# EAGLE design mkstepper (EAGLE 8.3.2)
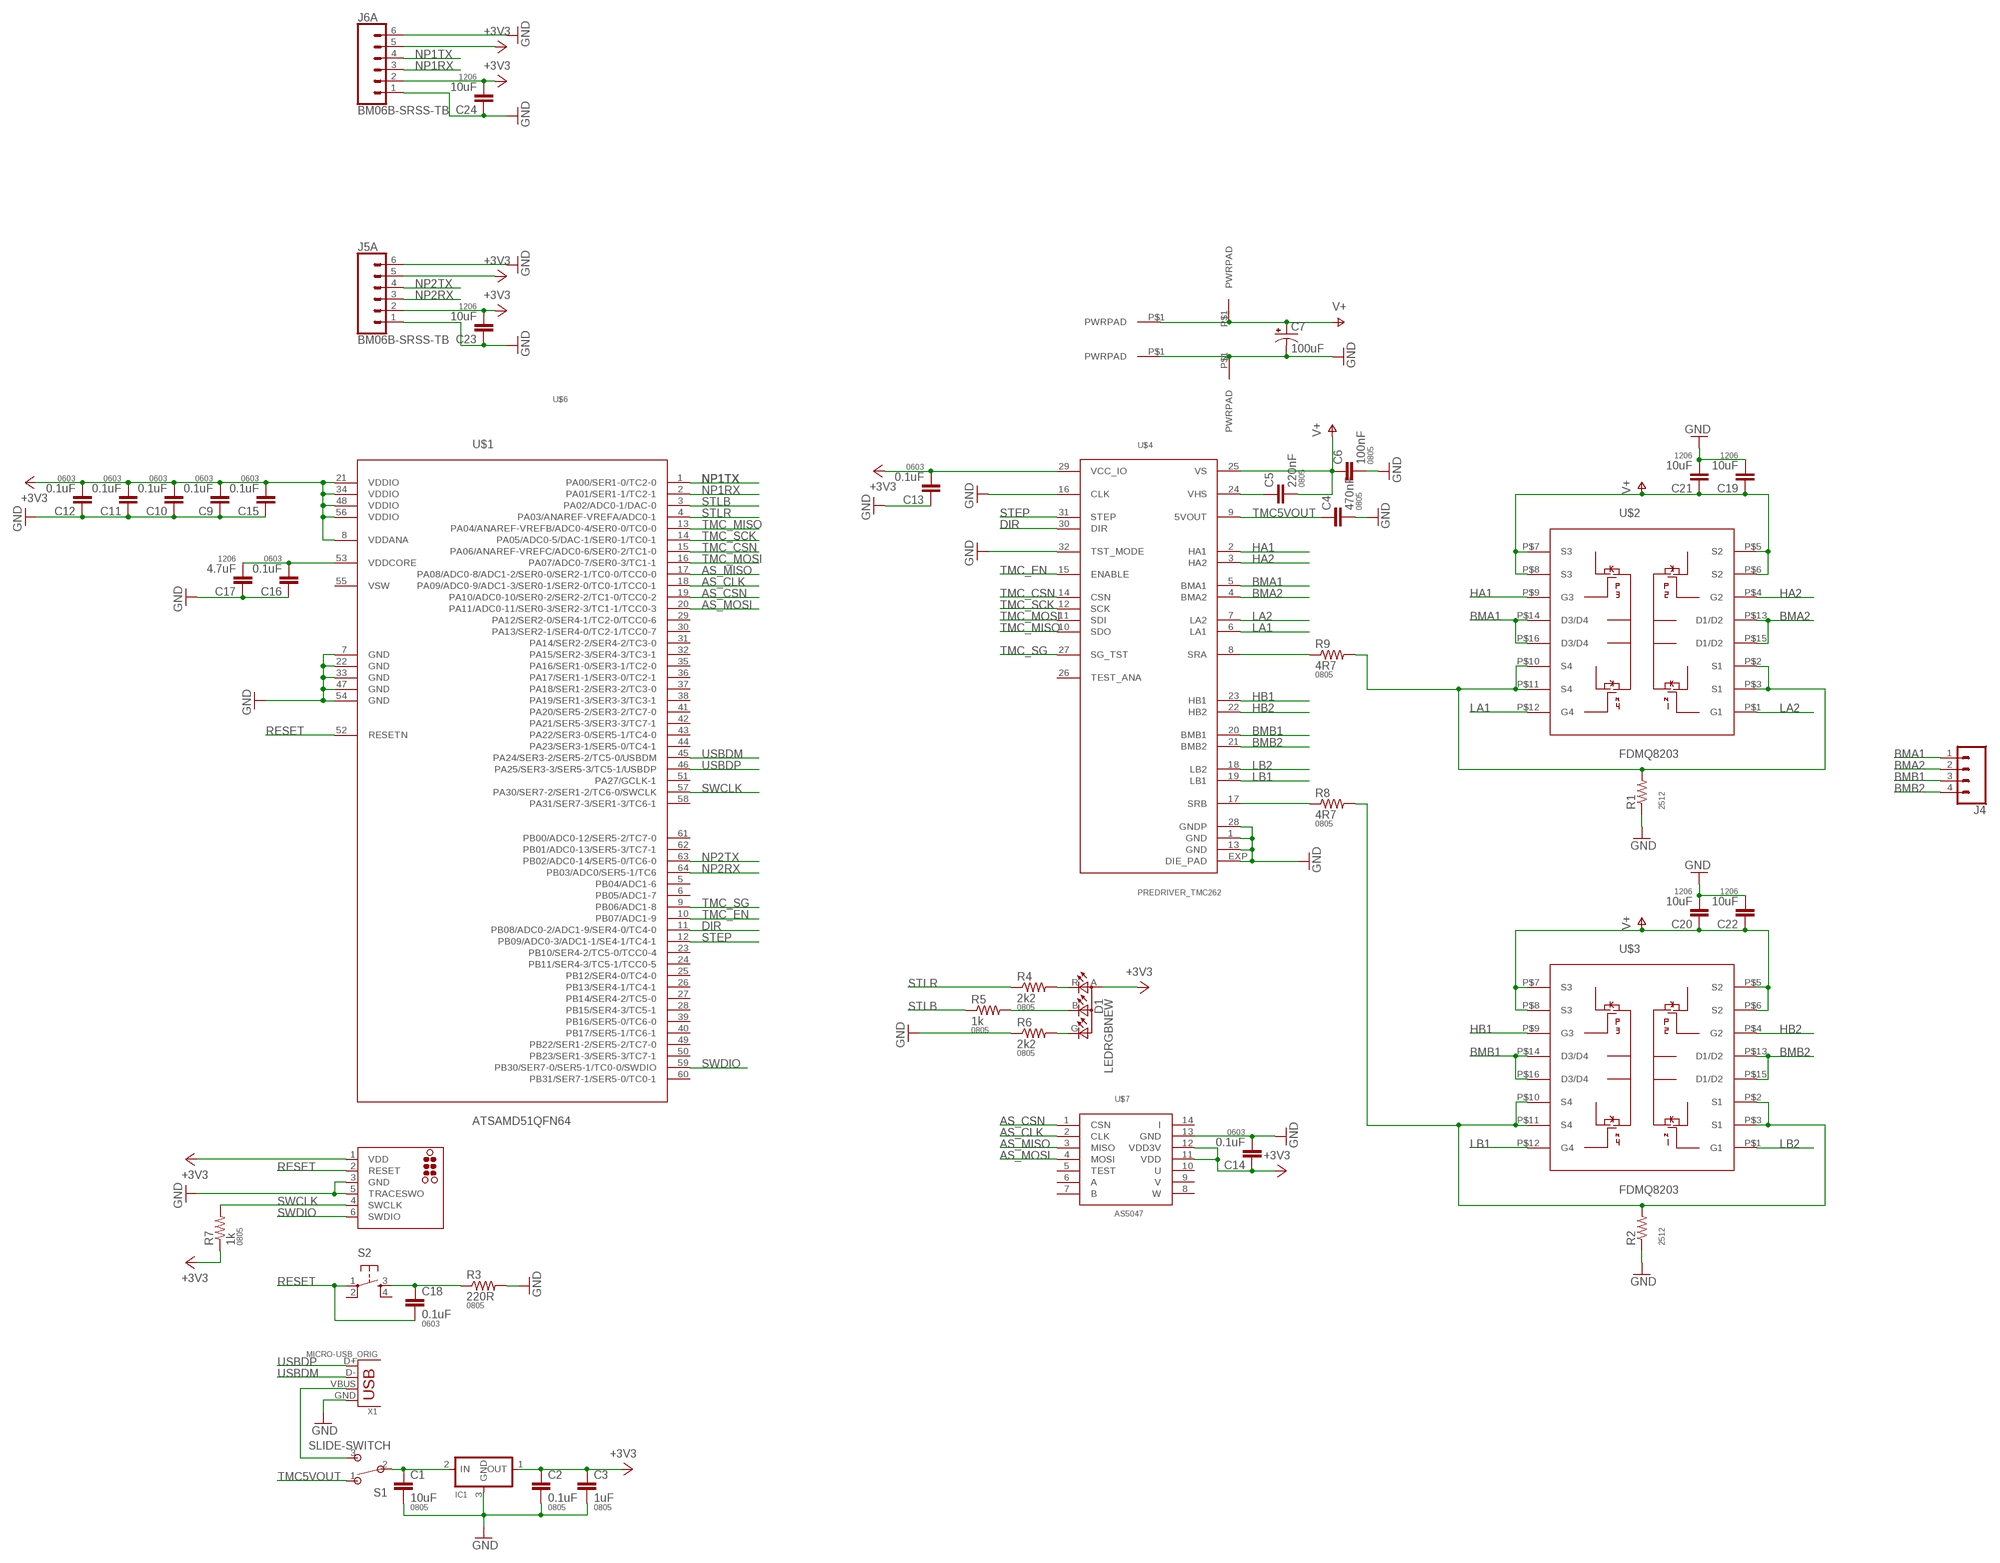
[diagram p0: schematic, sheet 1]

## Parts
C1  10uF  CAP0805  [0805]
C2  0.1uF  CAP0805  [0805]
C3  1uF  CAP0805  [0805]
C4  470nF  CAP0805  [0805]
C5  220nF  CAP0805  [0805]
C6  100nF  CAP0805  [0805]
C7  100uF  CAP-POL-6.6X6.6  [6.6X6.6-CAP]
C9  0.1uF  CAP0603-CAP  [0603-CAP]
C10  0.1uF  CAP0603-CAP  [0603-CAP]
C11  0.1uF  CAP0603-CAP  [0603-CAP]
C12  0.1uF  CAP0603-CAP  [0603-CAP]
C13  0.1uF  CAP0603-CAP  [0603-CAP]
C14  0.1uF  CAP0603-CAP  [0603-CAP]
C15  0.1uF  CAP0603-CAP  [0603-CAP]
C16  0.1uF  CAP0603-CAP  [0603-CAP]
C17  4.7uF  CAP1206  [1206]
C18  0.1uF  CAP0603-CAP  [0603-CAP]
C19  10uF  CAP1206  [1206]
C20  10uF  CAP1206  [1206]
C21  10uF  CAP1206  [1206]
C22  10uF  CAP1206  [1206]
C23  10uF  CAP1206  [1206]
C24  10uF  CAP1206  [1206]
D1  LEDRGBNEW  [P-LCC-4]
IC1  REGULATORSOT23  [SOT23]
J1  TC2030-SWD-MCP  [TC2030-MCP]
J2  PWRPAD2-5MM  [PWRPAD_2-5MM]
J3  PWRPAD2-5MM  [PWRPAD_2-5MM]
J4  CONN_04LONGPADS  [1X04_LONGPADS]
J5  BM06B-SRSS-TB  JST_6_PIN_HORIZONTAL  [JST-6-SMD-HORI-1.0MM]
J6  BM06B-SRSS-TB  JST_6_PIN_HORIZONTAL  [JST-6-SMD-HORI-1.0MM]
J7  PWRPAD2-5MM  [PWRPAD_2-5MM]
J9  PWRPAD2-5MM  [PWRPAD_2-5MM]
R1  RESISTOR2512  [R2512]
R2  RESISTOR2512  [R2512]
R3  220R  RESISTOR0805-RES  [0805]
R4  2k2  RESISTOR0805-RES  [0805]
R5  1k  RESISTOR0805-RES  [0805]
R6  2k2  RESISTOR0805-RES  [0805]
R7  1k  RESISTOR0805-RES  [0805]
R8  4R7  RESISTOR0805-RES  [0805]
R9  4R7  RESISTOR0805-RES  [0805]
S1  SLIDE-SWITCH  [AYZ0102AGRLC]
S2  6MM_SWITCH6MM_SWITCH  [6MM_SWITCH]
U$1  ATSAMD51QFN64  [QFN-64-9X9MM]
U$2  FDMQ8203  [MLP4.5X5_4PAD]
U$3  FDMQ8203  [MLP4.5X5_4PAD]
U$4  PREDRIVER_TMC262  [QFN32]
U$6  NEMA17  [NEMA17]
U$7  AS5047  [TSSOP14]
X1  MICRO-USB_ORIG  [DX4R005HJ5]

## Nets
+3V3: C2.1 C3.1 C9.2 C10.2 C11.2 C12.2 C13.2 C14.1 C15.2 C23.2 C24.2 D1.A(A2) IC1.1(OUT) J1.1(VDD) J5.2 J5.5 J6.2 J6.5 R7.1 U$1.8(VDDANA) U$1.21(VDDIO) U$1.34(VDDIO) U$1.48(VDDIO) U$1.56(VDDIO) U$4.29(VCC_IO) U$7.11(VDD) U$7.12(VDD3V)
AS_CLK: U$1.18(PA09/ADC0-9/ADC1-3/SER0-1/SER2-0/TC0-1/TCC0-1) U$7.2(CLK)
AS_CSN: U$1.19(PA10/ADC0-10/SER0-2/SER2-2/TC1-0/TCC0-2) U$7.1(CSN)
AS_MISO: U$1.17(PA08/ADC0-8/ADC1-2/SER0-0/SER2-1/TC0-0/TCC0-0) U$7.3(MISO)
AS_MOSI: U$1.20(PA11/ADC0-11/SER0-3/SER2-3/TC1-1/TCC0-3) U$7.4(MOSI)
BMA1: J4.1 U$2.P$14(D3/D4) U$2.P$16(D3/D4) U$4.5(BMA1)
BMA2: J4.2 U$2.P$13(D1/D2) U$2.P$15(D1/D2) U$4.4(BMA2)
BMB1: J4.3 U$3.P$14(D3/D4) U$3.P$16(D3/D4) U$4.20(BMB1)
BMB2: J4.4 U$3.P$13(D1/D2) U$3.P$15(D1/D2) U$4.21(BMB2)
DIR: U$1.11(PB08/ADC0-2/ADC1-9/SER4-0/TC4-0) U$4.30(DIR)
GND: C1.2 C2.2 C3.2 C4.2 C6.2 C7.- C9.1 C10.1 C11.1 C12.1 C13.1 C14.2 C15.1 C16.1 C17.1 C19.2 C20.2 C21.2 C22.2 C23.1 C24.1 IC1.3(GND) J1.3(GND) J1.5(TRACESWO) J3.P$1(PWRPAD) J5.1 J5.6 J6.1 J6.6 J7.P$1(PWRPAD) R1.1 R2.1 R3.2 R6.1 U$1.7(GND) U$1.22(GND) U$1.33(GND) U$1.47(GND) U$1.54(GND) U$4.1(GND) U$4.13(GND) U$4.16(CLK) U$4.28(GNDP) U$4.32(TST_MODE) U$4.EXP(DIE_PAD) U$7.13(GND) X1.GND
HA1: U$2.P$9(G3) U$4.2(HA1)
HA2: U$2.P$4(G2) U$4.3(HA2)
HB1: U$3.P$9(G3) U$4.23(HB1)
HB2: U$3.P$4(G2) U$4.22(HB2)
LA1: U$2.P$12(G4) U$4.6(LA1)
LA2: U$2.P$1(G1) U$4.7(LA2)
LB1: U$3.P$12(G4) U$4.19(LB1)
LB2: U$3.P$1(G1) U$4.18(LB2)
N$1: D1.G(CGREEN) R6.2
N$2: C5.1 U$4.24(VHS)
N$3: C1.1 IC1.2(IN) S1.2
N$4: S1.3 X1.VBUS
N$5: D1.B(CBLUE) R5.2
N$6: D1.R(CRED) R4.2
N$7: C16.2 C17.2 U$1.53(VDDCORE)
N$8: C18.1 R3.1 S2.3(S)
N$9: R2.2 R8.2 U$3.P$2(S1) U$3.P$3(S1) U$3.P$10(S4) U$3.P$11(S4)
N$10: R9.1 U$4.8(SRA)
N$11: R8.1 U$4.17(SRB)
N$12: R1.2 R9.2 U$2.P$2(S1) U$2.P$3(S1) U$2.P$10(S4) U$2.P$11(S4)
NP1RX: J6.3 U$1.2(PA01/SER1-1/TC2-1)
NP1TX: J6.4 U$1.1(PA00/SER1-0/TC2-0)
NP2RX: J5.3 U$1.64(PB03/ADC0/SER5-1/TC6)
NP2TX: J5.4 U$1.63(PB02/ADC0-14/SER5-0/TC6-0)
RESET: C18.2 J1.2(RESET) S2.1(P) U$1.52(RESETN)
STEP: U$1.12(PB09/ADC0-3/ADC1-1/SE4-1/TC4-1) U$4.31(STEP)
STLB: R5.1 U$1.3(PA02/ADC0-1/DAC-0)
STLR: R4.1 U$1.4(PA03/ANAREF-VREFA/ADC0-1)
SWCLK: J1.4(SWCLK) R7.2 U$1.57(PA30/SER7-2/SER1-2/TC6-0/SWCLK)
SWDIO: J1.6(SWDIO) U$1.59(PB30/SER7-0/SER5-1/TC0-0/SWDIO)
TMC5VOUT: C4.1 S1.1 U$4.9(5VOUT)
TMC_CSN: U$1.15(PA06/ANAREF-VREFC/ADC0-6/SER0-2/TC1-0) U$4.14(CSN)
TMC_EN: U$1.10(PB07/ADC1-9) U$4.15(ENABLE)
TMC_MISO: U$1.13(PA04/ANAREF-VREFB/ADC0-4/SER0-0/TC0-0) U$4.10(SDO)
TMC_MOSI: U$1.16(PA07/ADC0-7/SER0-3/TC1-1) U$4.11(SDI)
TMC_SCK: U$1.14(PA05/ADC0-5/DAC-1/SER0-1/TC0-1) U$4.12(SCK)
TMC_SG: U$1.9(PB06/ADC1-8) U$4.27(SG_TST)
USBDM: U$1.45(PA24/SER3-2/SER5-2/TC5-0/USBDM) X1.D-
USBDP: U$1.46(PA25/SER3-3/SER5-3/TC5-1/USBDP) X1.D+
V+: C5.2 C6.1 C7.+ C19.1 C20.1 C21.1 C22.1 J2.P$1(PWRPAD) J9.P$1(PWRPAD) U$2.P$5(S2) U$2.P$6(S2) U$2.P$7(S3) U$2.P$8(S3) U$3.P$5(S2) U$3.P$6(S2) U$3.P$7(S3) U$3.P$8(S3) U$4.25(VS)
Unconnected: J5.M1 J5.M2 J6.M1 J6.M2 S2.2(P1) S2.4(S1) U$1.5(PB04/ADC1-6) U$1.6(PB05/ADC1-7) U$1.23(PB10/SER4-2/TC5-0/TCC0-4) U$1.24(PB11/SER4-3/TC5-1/TCC0-5) U$1.25(PB12/SER4-0/TC4-0) U$1.26(PB13/SER4-1/TC4-1) U$1.27(PB14/SER4-2/TC5-0) U$1.28(PB15/SER4-3/TC5-1) U$1.29(PA12/SER2-0/SER4-1/TC2-0/TCC0-6) U$1.30(PA13/SER2-1/SER4-0/TC2-1/TCC0-7) U$1.31(PA14/SER2-2/SER4-2/TC3-0) U$1.32(PA15/SER2-3/SER4-3/TC3-1) U$1.35(PA16/SER1-0/SER3-1/TC2-0) U$1.36(PA17/SER1-1/SER3-0/TC2-1) U$1.37(PA18/SER1-2/SER3-2/TC3-0) U$1.38(PA19/SER1-3/SER3-3/TC3-1) U$1.39(PB16/SER5-0/TC6-0) U$1.40(PB17/SER5-1/TC6-1) U$1.41(PA20/SER5-2/SER3-2/TC7-0) U$1.42(PA21/SER5-3/SER3-3/TC7-1) U$1.43(PA22/SER3-0/SER5-1/TC4-0) U$1.44(PA23/SER3-1/SER5-0/TC4-1) U$1.49(PB22/SER1-2/SER5-2/TC7-0) U$1.50(PB23/SER1-3/SER5-3/TC7-1) U$1.51(PA27/GCLK-1) U$1.55(VSW) U$1.58(PA31/SER7-3/SER1-3/TC6-1) U$1.60(PB31/SER7-1/SER5-0/TC0-1) U$1.61(PB00/ADC0-12/SER5-2/TC7-0) U$1.62(PB01/ADC0-13/SER5-3/TC7-1) U$4.26(TEST_ANA) U$7.5(TEST) U$7.6(A) U$7.7(B) U$7.8(W) U$7.9(V) U$7.10(U) U$7.14(I)

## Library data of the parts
C1-C6 = borkedlabs-passives:CAP: Capacitor; PACKAGE: 0805
C7 = borkedlabs-passives:CAP-POL
C9-C16 C18 = borkedlabs-passives:CAP: Capacitor; PACKAGE: 0603
C17 C19-C24 = borkedlabs-passives:CAP: Capacitor; PACKAGE: 1206
D1 = fab:LEDRGBNEW
IC1 = fab:REGULATOR
J1 = atsam:TC2030-SWD: TAG-CONNECT ICSP Connector Manufacturer: Tag-Connect Cable for easy In-Circuit Serial Programming. Designed for Microchip ICD2, suitable for many others. Two variants - one "with legs" (for hands-free fit on PCB) and another "without legs" for quick programming. PADDescription 1MCLR/Vpp 2Vdd 3GND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
J2 J3 J7 J9 = power:PWRPAD
J4 = SparkFun-Connectors:CONN_04: Multi connection point. Often used as Generic Header-pin footprint for 0.1 inch spaced/style header connections On any of the 0.1 inch spaced packages, you can populate with these: Break Away Headers - Straight (PRT-00116) Break Away Male Headers - Right Angle (PRT-00553) Female Headers (PRT-00115)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; PROD_ID: CONN-09696
J5 J6 = SparkFun-Connectors:JST_6_PIN_HORIZONTAL: JST 6 pin horizontal connector JST-SH type. Here is the connector we sell at SparkFun: name (XXX-00000) Datasheet It was used on these SparkFun products: name (XXX-00000) name (XXX-00000); PROD_ID: XXX-00000
R1 R2 = borkedlabs-passives:RESISTOR: Resistor; PACKAGE: 2512
R3-R9 = borkedlabs-passives:RESISTOR: Resistor; PACKAGE: 0805
S1 = fab:SLIDE-SWITCH: SMD slide-switch AYZ0102AGRLC as found in the fablab inventory. Includes the mounting holes. Made by Zaerc.
S2 = fab:6MM_SWITCH: OMRON SWITCH
U$1 = atsam:ATSAMD51
U$2 U$3 = power:FDMQ8203
U$4 = power:PREDRIVER_TMC262
U$6 = motors:NEMA17
U$7 = sensor:AS5047
X1 = fab:MICRO-USB: SMD micro USB connector as found in the fablab inventory. Three footprint variants included: original, as described by manufacturer's datasheet for milling with the 1/100" bit for milling with the 1/64" bit Made by Zaerc.

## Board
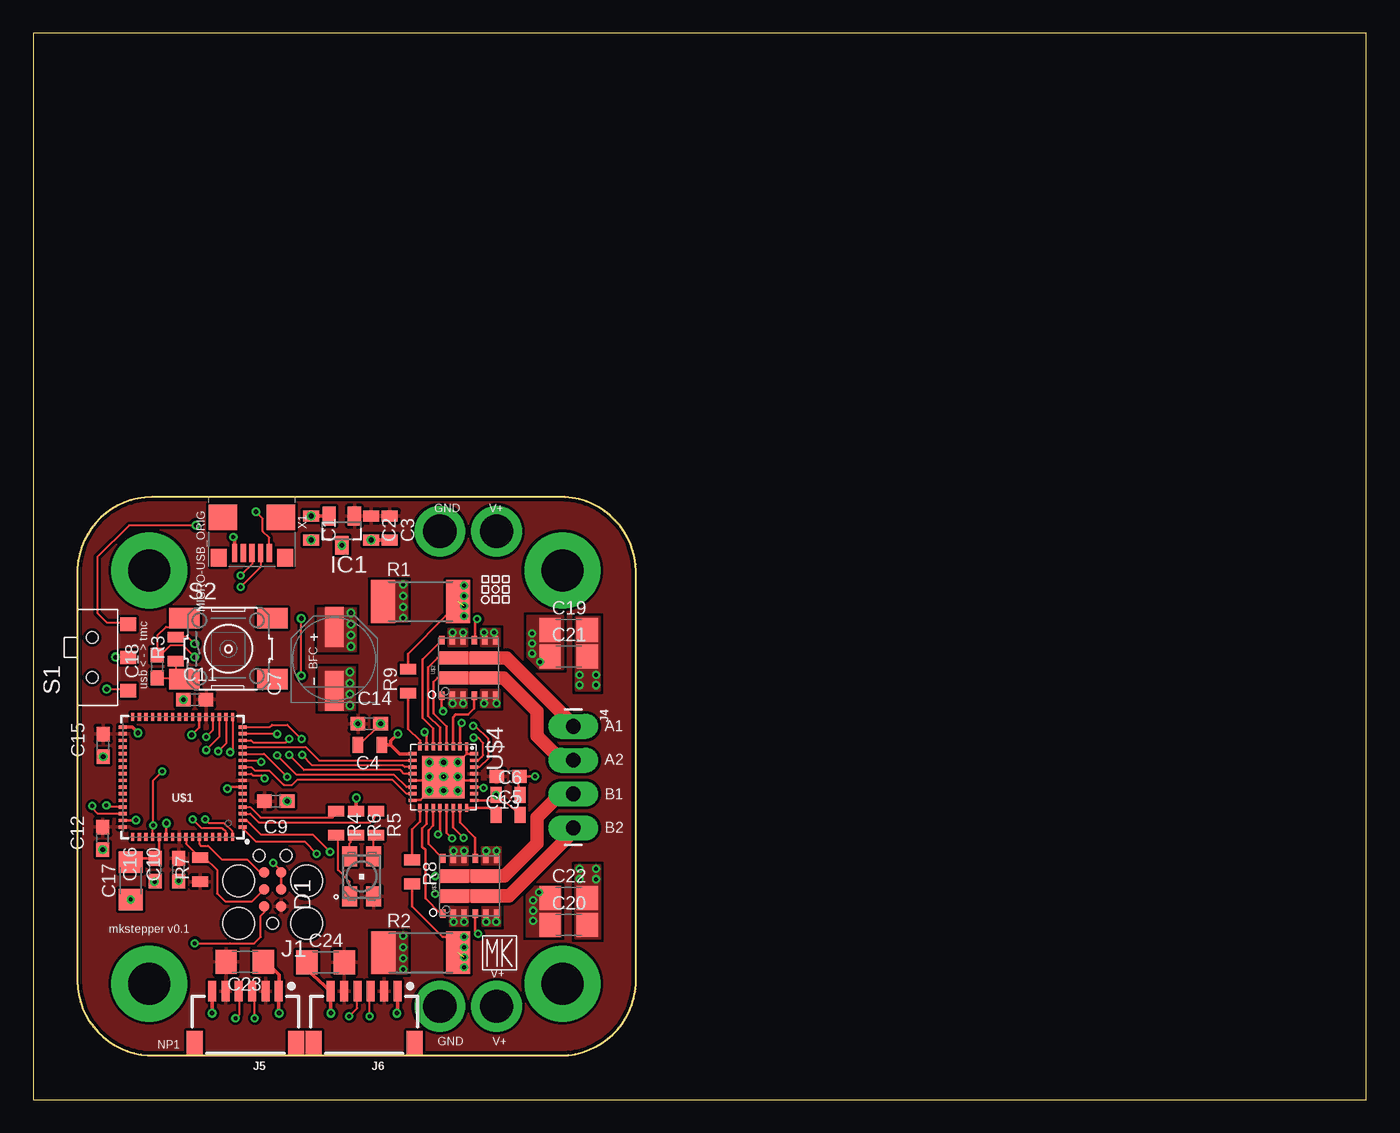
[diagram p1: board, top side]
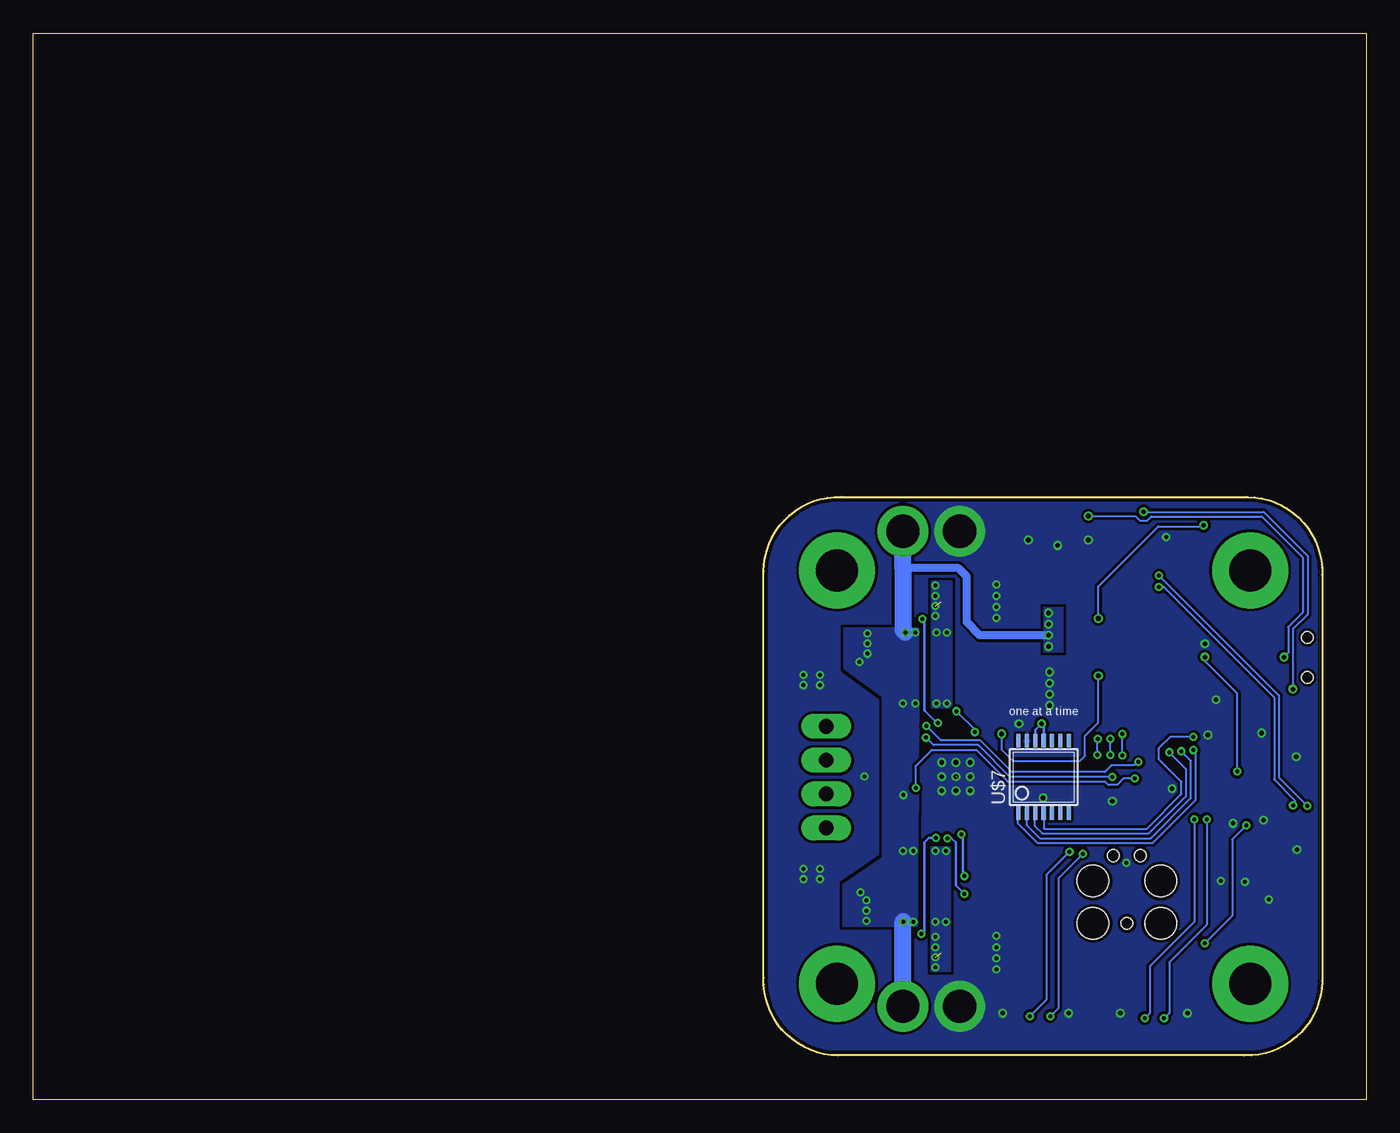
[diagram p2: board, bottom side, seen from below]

Size 100 x 80 mm. Coordinates in mm from the lower left corner, seen from the top.
Outline: 0,0 100,0 100,80 0,80 0,0
Outline: 8.89,45.21 arc91 3.3,39.37 3.3,8.89 arc91 9.14,3.3 39.62,3.3 arc91 45.21,9.14 45.21,39.62 arc91 39.37,45.21 8.89,45.21
Copper layers (1*16): Top 0.035mm / dielectric 1.5mm / Bottom 0.035mm
Design rules "default *": minimum track width 6mil, minimum drill 0.3mm, track to track 8mil, track to pad 8mil, pad to pad 8mil, via to via 8mil, smd to smd 8mil, copper to edge 10mil, drill to drill 10mil, minimum pad ring 6mil, minimum via ring 6mil, stop-mask expansion 4mil, vias tented up to drill 27mil, thermal gap 9mil

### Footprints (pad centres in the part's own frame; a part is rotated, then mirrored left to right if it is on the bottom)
0805 = smd 0.8 x 1.2: 1 -0.9,0; 2 0.9,0
6.6X6.6-CAP = smd 3 x 1.4: + 2.4,0; - -2.4,0
0603-CAP = smd 1.1 x 1: 1 -0.85,0; 2 0.85,0
1206 = smd 1.6 x 1.8: 1 -1.4,0; 2 1.4,0
P-LCC-4 = smd 1.1 x 1.5: A 0.902,-1.5; B 0.902,1.5; G -0.902,1.5; R -0.902,-1.5
SOT23 = smd 1 x 1.4: 1 -0.95,-1.1; 2 0.95,-1.1; 3 0,1.1
TC2030-MCP = smd 0.787 x 0.787: 1 1.27,-0.635; 2 1.27,0.635; 3 2.54,-0.635; 4 2.54,0.635; 5 3.81,-0.635; 6 3.81,0.635 | hole 0.889: 0,0; 5.08,-1.016; 5.08,1.016 | hole 2.375: 0,2.54; 0,-2.54; 3.175,-2.54; 3.175,2.54
PWRPAD_2-5MM = drill 2.489 pad 3.81: P$1 0,0
1X04_LONGPADS = drill 1.118 pad 1.88 long: 1 0,0; 2 2.54,0; 3 5.08,0; 4 7.62,0
JST-6-SMD-HORI-1.0MM = smd 0.6 x 1.55: 1 -2.5,-4.775; 2 -1.5,-4.775; 3 -0.5,-4.775; 4 0.5,-4.775; 5 1.5,-4.775; 6 2.5,-4.775 | smd 1.2 x 1.8: M1 -3.8,-0.9; M2 3.8,-0.9
R2512 = smd 1.8 x 3.2: 1 -2.8,0; 2 2.8,0
AYZ0102AGRLC = smd 1 x 1.2: 1 2.5,-2.3; 2 0,-2.3; 3 -2.5,-2.3 | hole 0.85: -1.5,0.4; 1.5,0.4
6MM_SWITCH = smd 2.286 x 1.524: 1 -3.302,2.286; 2 3.302,2.286; 3 -3.302,-2.286; 4 3.302,-2.286
QFN-64-9X9MM = smd 0.6 x 0.25: 1 -4.5,3.75; 2 -4.5,3.25; 3 -4.5,2.75; 4 -4.5,2.25; 5 -4.5,1.75; 6 -4.5,1.25; 7 -4.5,0.75; 8 -4.5,0.25; 9 -4.5,-0.25; 10 -4.5,-0.75; 11 -4.5,-1.25; 12 -4.5,-1.75; 13 -4.5,-2.25; 14 -4.5,-2.75; 15 -4.5,-3.25; 16 -4.5,-3.75; 33 4.5,-3.75; 34 4.5,-3.25; 35 4.5,-2.75; 36 4.5,-2.25; 37 4.5,-1.75; 38 4.5,-1.25; 39 4.5,-0.75; 40 4.5,-0.25; 41 4.5,0.25; 42 4.5,0.75; 43 4.5,1.25; 44 4.5,1.75; 45 4.5,2.25; 46 4.5,2.75; 47 4.5,3.25; 48 4.5,3.75 | smd 0.25 x 0.6: 17 -3.75,-4.5; 18 -3.25,-4.5; 19 -2.75,-4.5; 20 -2.25,-4.5; 21 -1.75,-4.5; 22 -1.25,-4.5; 23 -0.75,-4.5; 24 -0.25,-4.5; 25 0.25,-4.5; 26 0.75,-4.5; 27 1.25,-4.5; 28 1.75,-4.5; 29 2.25,-4.5; 30 2.75,-4.5; 31 3.25,-4.5; 32 3.75,-4.5; 49 3.75,4.5; 50 3.25,4.5; 51 2.75,4.5; 52 2.25,4.5; 53 1.75,4.5; 54 1.25,4.5; 55 0.75,4.5; 56 0.25,4.5; 57 -0.25,4.5; 58 -0.75,4.5; 59 -1.25,4.5; 60 -1.75,4.5; 61 -2.25,4.5; 62 -2.75,4.5; 63 -3.25,4.5; 64 -3.75,4.5
MLP4.5X5_4PAD = smd 0.4 x 0.65: P$1 -2.02,-2.075; P$2 -1.22,-2.075; P$3 -0.42,-2.075; P$4 0.42,-2.075; P$5 1.22,-2.075; P$6 2.02,-2.075; P$7 2.02,2.075; P$8 1.22,2.075; P$9 0.42,2.075; P$10 -0.42,2.075; P$11 -1.22,2.075; P$12 -2.02,2.075 | smd 2.1 x 1: P$13 1.142,-0.75; P$14 1.142,0.75; P$15 -1.142,-0.75; P$16 -1.142,0.75
QFN32 = smd 0.6 x 0.25: 1 -2.3,1.75; 2 -2.3,1.25; 3 -2.3,0.75; 4 -2.3,0.25; 5 -2.3,-0.25; 6 -2.3,-0.75; 7 -2.3,-1.25; 8 -2.3,-1.75; 17 2.3,-1.75; 18 2.3,-1.25; 19 2.3,-0.75; 20 2.3,-0.25; 21 2.3,0.25; 22 2.3,0.75; 23 2.3,1.25; 24 2.3,1.75 | smd 0.25 x 0.6: 9 -1.75,-2.3; 10 -1.25,-2.3; 11 -0.75,-2.3; 12 -0.25,-2.3; 13 0.25,-2.3; 14 0.75,-2.3; 15 1.25,-2.3; 16 1.75,-2.3; 25 1.75,2.3; 26 1.25,2.3; 27 0.75,2.3; 28 0.25,2.3; 29 -0.25,2.3; 30 -0.75,2.3; 31 -1.25,2.3; 32 -1.75,2.3 | smd 3.2 x 3.2: EXP 0,0
NEMA17 = drill 3.15 pad 5.7: P$1 -15.5,15.5; P$2 15.5,15.5; P$3 -15.5,-15.5; P$4 15.5,-15.5
TSSOP14 = smd 0.305 x 0.991: 1 -1.905,-2.718; 2 -1.27,-2.718; 3 -0.635,-2.718; 4 0,-2.718; 5 0.635,-2.718; 6 1.27,-2.718; 7 1.905,-2.718; 8 1.905,2.718; 9 1.27,2.718; 10 0.635,2.718; 11 0,2.718; 12 -0.635,2.718; 13 -1.27,2.718; 14 -1.905,2.718
DX4R005HJ5 = smd 0.4 x 1.35: D+ 0,1.6; D- -0.65,1.6; GND 1.3,1.6; ID 0.65,1.6; VBUS -1.3,1.6 | smd 1.2 x 1.3: GND@1 -2.5,1.95; GND@2 2.5,1.95 | smd 2.15 x 1.9: GND@3 -2.175,-1.1; GND@4 2.175,-1.1

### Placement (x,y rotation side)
C1  20.84,42.88 270 top
C2  25.34,42.88 270 top
C3  26.74,42.88 270 top
C4  25.24,26.61 180 top
C5  35.62,21.36 0 top
C6  35.62,22.84 0 top
C7  22.59,33.04 90 top
C9  18.2,22.38 180 top
C10  10.9,17.25 90 top
C11  12.11,30 0 top
C12  5.2,19.6 90 top
C13  35.62,24.24 180 top
C14  25.2,28.2 0 top
C15  5.24,26.57 90 top
C16  9.15,17.25 90 top
C17  7.3,16.4 90 top
C18  9.3,32.49 90 top
C19  40.17,35.25 0 top
C20  40.17,13.1 0 top
C21  40.17,33.25 0 top
C22  40.17,15.14 0 top
C23  15.87,10.32 180 top
C24  21.93,10.3 0 top
D1  24.63,16.74 0 top
IC1  23.14,42.68 180 top
J1  17.95,13.22 90 top
J2  34.75,42.64 0 top
J3  30.5,42.64 0 top
J4  40.51,28 270 top
J5  15.92,3.35 180 top
J6  24.82,3.35 180 top
J7  30.5,7 0 top
J9  34.75,7 0 top
R1  29.06,37.37 0 top
R2  29.07,11.01 0 top
R3  10.67,33.79 90 top
R4  22.74,20.73 270 top
R5  25.73,20.73 270 top
R6  24.23,20.73 270 top
R7  12.5,17.25 90 top
R8  28.41,17.08 270 top
R9  28.11,31.38 90 top
S1  4.82,33.17 90 top
S2  14.63,33.82 0 top
U$1  11.2,24.2 180 top
U$2  32.67,32.38 0 top
U$3  32.74,16.02 0 top
U$4  30.75,24.19 270 top
U$5  [CBA-SILK-LOGO]  34.68,38.27 90 top
U$6  24.2,24.2 0 top
U$7  24.2,24.2 0 bottom
U$9  [MK-LOGO-SILK]  34.98,11.01 0 top
X1  16.4,42.6 180 top

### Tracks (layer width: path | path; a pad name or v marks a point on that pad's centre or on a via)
+3V3  (via drill 0.35)
  Bottom 0.203: U$7.11 24.2,28.05 C14.1 24.84,27.71 U$7.12
  other vias: 24.35,28.2
  pour Top (rank 2): 3.15,39.65 3.3,45.21 8.7,45.2 39.7,45.2 45.21,45.21 45.25,39.65 45.25,8.7 45.21,3.3 39.7,3.15 8.7,3.15 3.3,3.3 3.15,8.7
AS_CLK  (via drill 0.3)
  Top 0.152: U$1.18 14.45,26.72 v13.87,26.14
  Bottom 0.152: U$7.2 25.45,21.46 25.45,20.57 24.49,19.61 16.16,19.61 13.14,22.63 13.14,25.41 v13.87,26.14
AS_CSN  (via drill 0.3)
  Top 0.152: U$1.19 13.95,27.21 v12.95,26.21
  Bottom 0.152: U$7.1 26.14,21.45 26.14,20.73 24.66,19.25 16.01,19.25 12.79,22.48 12.79,26.05 v12.95,26.21
AS_MISO  (via drill 0.3)
  Top 0.152: U$1.17 14.95,26.23 v14.78,26.06
  Bottom 0.152: U$7.3 24.84,20.5 24.31,19.96 16.31,19.96 13.5,22.77 13.5,24.77 v14.78,26.06
AS_MOSI  (via drill 0.3)
  Top 0.152: U$1.20 13.45,27.7 v12.95,27.2
  Bottom 0.152: v12.95,27.2 14.71,27.2 15.54,26.36 15.54,25.53 13.85,23.84 13.85,22.92 16.45,20.32 24.16,20.32 24.2,20.36 U$7.4
BMA1
  Top 0.203: U$4.5 30.5,27.9 29.62,28.79 29.62,32.44 30.33,33.15 31.51,33.15 U$2.P$16
  Top 1.016: U$2.P$16 U$2.P$14 35.52,33.13 40.08,28.57 40.08,28.43 J4.1
BMA2
  Top 0.203: U$4.4 31,27.98 30.02,28.96 30.02,31.32 30.33,31.62 U$2.P$15
  Top 1.016: U$2.P$15 U$2.P$13 35.27,31.63 37.8,29.11 37.8,27.28 39.55,25.53 40.45,25.53 J4.2
BMB1  (via drill 0.3)
  Top 0.203: U$4.20 30.5,20.02 v30.37,19.89 | v30.14,16.76 U$3.P$16
  Top 1.016: J4.3 40.45,22.86 39.47,22.86 37.8,21.18 37.8,19.2 35.36,16.77 U$3.P$14 U$3.P$16
  Bottom 0.203: v30.37,19.89 30.37,19.86 30.25,19.74 30.25,16.88 v30.14,16.76
BMB2  (via drill 0.3)
  Top 0.203: U$4.21 31,20.01 v31.42,19.6 | v30.14,15.42 31.44,15.42 U$3.P$15
  Top 1.016: J4.4 40.23,20.1 40.23,19.81 35.69,15.27 U$3.P$13 U$3.P$15
  Bottom 0.203: v31.42,19.6 31.1,19.6 30.79,19.28 30.79,16.07 v30.14,15.42
DIR  (via drill 0.3)
  Top 0.152: U$1.11 16.95,25.45 v17.09,25.32 | v33,28.04 33.15,28.04 34.14,27.05 34.14,25.6 33.47,24.94 U$4.30
  Bottom 0.152: v17.09,25.32 17.2,25.32 17.45,25.07 19.13,25.07 19.62,24.58 26.59,24.58 28.96,26.95 31.9,26.95 v33,28.04
GND  (via drill 0.3, 0.35)  (1 unrouted)
  Top 0.152: R3.2 11.51,34.79 v12.1,34.2
  Top 0.203: U$4.13 30.5,23.94 U$4.EXP | U$4.16 28.7,22.44 28.75,22.49 29.06,22.49 U$4.EXP | U$4.28 31,23.94 U$4.EXP | 32.5,25.94 U$4.32 | 32.5,25.94 U$4.EXP | U$4.1 32.5,25.94 | C6.2 36.29,24.19 C13.1 37.41,24.24 v37.64,24.23 | C16.1 v9.09,16.34 | U$1.54 9.95,20.69 v9.98,20.73 | U$1.47 v7.69,20.95 v7.7,20.95 | U$1.7 14.69,23.45 v14.55,23.32 | C4.2 24.46,26.61 C14.2 | v17.98,17.75 18.59,17.15 J1.5 J1.3 | U$1.22 12.45,27.92 v11.89,27.36
  Top 0.254: X1.GND 15.1,42.13 v15.01,42.22 | U$1.33 7.41,27.95 v7.85,27.51 | C3.2 C2.2 | v18.44,6.48 18.42,6.49 J5.1 18.44,7.94 18.44,9.37 17.59,10.22 C23.1 | J5.6 13.42,6.49 v13.41,6.48 | v22.33,6.48 22.32,6.49 J6.6 20.53,9.72 C24.1 | J6.1 27.32,6.52 v27.28,6.48 | R6.1 v24.23,22.63
  other vias: 26.05,28.2 29.72,25.3 31.85,25.3 30.78,25.3 29.72,24.23 29.72,23.16 30.78,24.23 30.78,23.16 31.85,23.16 31.85,24.23 27.74,38.63 27.74,36.12 27.74,36.96 27.74,37.8 41,31.85 42.21,31.85 41,31.09 42.21,31.09 27.74,12.27 27.74,9.75 27.74,10.59 27.74,11.43 41,17.3 41,16.54 42.21,16.54 42.21,17.3 10.9,16.4 7.3,15 5.24,25.72 11.26,30 19.05,22.38 20.84,41.98 23.14,41.58 25.34,41.98 23.74,32.09 23.74,31.25 23.74,30.41 23.74,29.57 5.2,18.75
  pour Bottom (rank 2): 3.15,39.65 3.3,45.21 8.7,45.2 39.7,45.2 45.21,45.21 45.25,39.65 45.25,8.7 45.21,3.3 39.7,3.15 8.7,3.15 3.3,3.3 3.15,8.7
  pour Top (no thermals): 25.37,38.94 28.04,38.94 28.04,35.81 25.37,35.81
  pour Top (no thermals): 40.69,36.2 40.69,30.71 42.52,30.71 42.52,36.2
  pour Top (no thermals): 25.37,12.57 28.04,12.57 28.04,9.45 25.37,9.45
  pour Top (no thermals): 40.69,12.04 40.69,17.6 42.52,17.6 42.52,12.04
  pour Top (no thermals): 21.45,32.47 24.12,32.47 24.12,29.19 21.45,29.19
HA1  (via drill 0.3, 0.3 pad 0.42)
  Top 0.203: U$4.2 32,28.11 v32.14,28.25 | v33.3,36.04 33.15,35.89 33.15,34.52 U$2.P$9
  Bottom 0.203: v32.14,28.25 32.21,28.25 33.15,29.18 33.15,35.89 v33.3,36.04
HA2
  Top 0.203: U$2.P$4 33.09,29.35 32.61,28.88 31.7,28.88 31.5,28.68 U$4.3
HB1
  Top 0.203: U$4.23 32,20.8 33.16,19.64 U$3.P$9
HB2  (via drill 0.3)
  Top 0.203: U$4.22 31.5,20.41 v32.28,19.63 | v33.38,12.42 33.15,12.65 33.15,13.93 U$3.P$4
  Bottom 0.203: v32.28,19.63 32.79,19.63 33.15,19.28 33.15,12.65 v33.38,12.42
LA1
  Top 0.203: U$4.6 30,27.83 29.21,28.62 29.21,33.02 U$2.P$12
LA2  (via drill 0.3)
  Top 0.203: U$4.7 29.5,27.43 v29.37,27.56 | U$2.P$1 30.65,29.23 v30.74,29.14
  Bottom 0.203: v29.37,27.56 29.37,27.77 v30.74,29.14
LB1
  Top 0.203: U$4.19 30,20.55 29.64,20.19 29.64,19.17 U$3.P$12
LB2
  Top 0.203: U$4.18 29.5,20.66 29.18,20.34 29.18,18.97 29.41,18.75 29.41,15.09 30.56,13.94 U$3.P$1
N$1
  Top 0.152: D1.G 23.73,19.23 23.82,19.31 23.82,19.41 R6.2
N$2
  Top 0.203: U$4.24 34.19,21.89 C5.1
N$3  (via drill 0.35)
  Top 0.152: v6.16,33.2 7.09,33.2 S1.2
  Top 0.254: IC1.2 C1.1
  Bottom 0.152: C1.1 17.31,43.78 16.97,43.44 16.43,43.44 16.13,43.74 7.85,43.74 4.76,40.65 4.76,36.55 5.86,35.45 5.86,33.5 v6.16,33.2
  other vias: 20.84,43.78
N$4  (via drill 0.35)
  Top 0.152: v16.7,44.1 17.22,43.58 17.22,42.63 17.7,42.16 X1.VBUS | v5.5,30.8 7,30.8 S1.3
  Bottom 0.152: v16.7,44.1 7.7,44.1 4.4,40.8 4.4,36.4 5.5,35.3 v5.5,30.8
N$5
  Top 0.152: D1.B 25.54,19.82 R5.2
N$6
  Top 0.152: D1.R 23.73,16.35 22.86,17.22 22.86,19.75 R4.2
N$7
  Top 0.203: U$1.53 9.45,18.4 C16.2 7.6,18.1 C17.2
N$8
  Top 0.152: 11.18,31.68 11.02,31.84 10.67,32.18 R3.1 | 11.18,31.68 S2.3 | C18.1 11.14,31.64 11.18,31.68
N$9  (via drill 0.3)  (1 unrouted)
  Top 0.203: R8.2 28.41,14.49 30.71,12.19 v32.31,12.19
  other vias: 31.55,18.67 32.31,18.67 31.55,13.34 32.31,13.34 32.31,9.91 32.31,10.67 32.31,11.43
  pour Bottom: 31.24,18.97 31.24,9.6 32.61,9.6 32.61,18.97
  pour Top (no thermals): 31.24,18.97 31.24,17.6 32.61,17.6 32.61,18.97
  pour Top (no thermals): 31.24,13.03 32.61,13.03 32.61,14.48 31.24,14.48
N$10
  Top 0.203: U$4.8 29,26.93 28.12,27.81 28.12,28.95 R9.1
N$11
  Top 0.203: U$4.17 29,20.85 28.41,20.26 R8.1
N$12  (via drill 0.3, 0.3 pad 0.55)  (1 unrouted)
  Top 0.203: v32.31,36.27 30.94,36.27 28.11,33.45 R9.2
  other vias: 32.31,38.56 32.31,37.8 32.31,37.03 31.47,35.05 32.23,35.05 31.47,29.72 32.23,29.72
  pour Bottom: 31.09,29.41 31.09,38.86 32.61,38.86 32.61,29.41
  pour Top (no thermals): 31.17,33.99 31.17,35.36 32.54,35.36 32.54,33.99
  pour Top (no thermals): 31.17,30.78 31.17,29.41 32.54,29.41 32.54,30.78
NP1RX  (via drill 0.3)
  Top 0.152: U$1.2 16.02,20.95 16.28,20.69 16.28,20.68 17.07,19.89 20.95,19.89 v22.25,18.59 | v25.22,6.25 25.22,7.83 J6.3
  Bottom 0.152: v22.25,18.59 24,16.84 24,7.47 v25.22,6.25
NP1TX  (via drill 0.3)
  Top 0.152: U$1.1 15.7,20.34 16.69,19.36 20.34,19.36 v21.26,18.44 | v23.7,6.25 24.31,6.86 24.31,7.92 J6.4
  Bottom 0.152: v21.26,18.44 23.09,16.61 23.09,6.86 v23.7,6.25
NP2RX  (via drill 0.3)
  Top 0.152: U$1.64 14.95,20.1 14.33,20.73 13.18,20.73 v12.88,21.03 | v16.61,6.1 16.61,7.74 J5.3
  Bottom 0.152: v12.88,21.03 12.88,13.34 16.23,9.98 16.23,6.48 v16.61,6.1
NP2TX  (via drill 0.3)
  Top 0.152: U$1.63 14.45,20.07 14.17,20.34 12.65,20.34 v11.96,21.03 | v15.16,6.1 15.47,6.4 15.47,7.88 J5.4
  Bottom 0.152: v11.96,21.03 11.96,13.11 14.78,10.29 14.78,6.48 v15.16,6.1
RESET  (via drill 0.3, 0.35)
  Top 0.152: J1.2 17.32,14.04 17.07,13.79 17.07,12.19 16.58,11.7 14.78,11.7 14.75,11.73 v12.12,11.73 | U$1.52 8.95,20.53 v8.99,20.57 8.99,23.93 v9.68,24.61 | 11.49,36.27 S2.1 11.33,35.95 10.85,35.47 9.96,35.47 9.3,34.8 C18.2 9.54,33.34 10.3,34.1 11.2,34.1 v12.1,33.2
  Bottom 0.152: v8.99,20.57 10.06,19.51 10.06,13.79 v12.12,11.73 | v12.1,33.2 12.1,32.9 9.68,30.48 v9.68,24.61
STEP  (via drill 0.3)
  Top 0.152: U$1.12 17.31,25.95 v19.04,24.22 | v33.02,27.15 33.35,27.15 33.76,26.75 33.76,25.83 33.63,25.71 33.63,25.7 33.37,25.44 U$4.31
  Bottom 0.152: v19.04,24.22 26.74,24.22 29.11,26.59 32.46,26.59 v33.02,27.15
STLB
  Top 0.152: R5.1 25.53,21.03 25.3,20.8 16.92,20.8 16.27,21.45 U$1.3
STLR
  Top 0.152: U$1.4 16.27,21.95 17.05,21.17 22.48,21.17 R4.1
SWCLK
  Top 0.152: U$1.57 11.45,19.2 R7.2 12.86,18.15 13.79,17.22 13.79,15.47 14.4,14.86 16.41,14.86 J1.4
SWDIO
  Top 0.152: J1.6 17.03,17.03 16.08,17.98 14.17,17.98 13.11,19.05 12.57,19.05 12.45,19.17 U$1.59
TMC5VOUT  (via drill 0.35)
  Top 0.152: v20.1,31.8 v20.1,36.1 | v12.2,43.09 7.19,43.09 4.8,40.7 4.8,36.5 5.5,35.8 7,35.8 S1.1
  Top 0.254: U$4.9 27.48,25.94 26.82,26.59 | 26.82,26.59 26.15,26.59 C4.1 | 26.82,26.59 26.82,26.9 v27.36,27.43
  Bottom 0.152: v27.36,27.43 27.36,26.26 26.5,25.4 21.5,25.4 21.1,25.8 21.1,27.3 20.1,28.3 v20.1,31.8 | v20.1,36.1 20.1,38.5 15.6,43 12.29,43 v12.2,43.09
TMC_CSN  (via drill 0.3)
  Top 0.152: U$4.14 28,23.44 27.06,24.37 19.75,24.37 v18.29,25.83 | v18.29,27.41 15.74,27.41 U$1.15
  Bottom 0.152: v18.29,25.83 v18.29,27.41
TMC_EN
  Top 0.152: U$4.15 27.99,22.94 26.92,24.02 19.82,24.02 19.42,23.61 18.79,23.61 17.71,24.69 16.61,24.69 16.35,24.95 U$1.10
TMC_MISO
  Top 0.152: U$1.13 20.41,26.45 21.43,25.44 U$4.10
TMC_MOSI  (via drill 0.3)
  Top 0.152: U$4.11 27.87,24.94 27.72,25.08 20.92,25.08 v20.16,25.84 | v20.12,27.06 v20.11,27.06 19.05,28.12 17.91,28.12 17.74,27.95 U$1.16
  Bottom 0.152: v20.16,25.84 20.16,27.01 v20.12,27.06
TMC_SCK  (via drill 0.3)
  Top 0.152: U$4.12 27.84,24.44 27.55,24.73 20.32,24.73 v19.2,25.84 | U$1.14 16.33,26.95 16.48,26.81 18.95,26.81 v19.2,27.06
  Bottom 0.152: v19.2,25.84 v19.2,27.06
TMC_SG  (via drill 0.3)
  Top 0.152: U$4.27 33.74,23.44 v33.79,23.39 | U$1.9 16.35,24.45 16.46,24.33 17.1,24.33 v17.35,24.08
  Bottom 0.152: v33.79,23.39 33.79,25.04 32.59,26.24 29.26,26.24 26.88,23.86 19.6,23.86 19.36,23.62 19.3,23.62 19.29,23.61 18.68,23.61 18.21,24.08 v17.35,24.08
USBDM  (via drill 0.3)
  Top 0.152: X1.D- 17.05,39.97 v15.54,38.46 | U$1.45 5.59,21.95 v5.49,22.06
  Bottom 0.152: v15.54,38.46 15.19,38.46 6.91,30.18 6.91,24.01 5.36,22.46 5.36,22.19 v5.49,22.06
USBDP  (via drill 0.3)
  Top 0.152: X1.D+ 16.4,40.17 v15.54,39.32 | v4.42,22.02 4.42,21.87 4.84,21.45 U$1.46
  Bottom 0.152: v4.42,22.02 6.55,24.16 6.55,30.33 v15.54,39.32
V+  (via drill 0.3, 0.3 pad 0.42, 0.35)
  Top 0.203: C5.2 34.81,22.84 C6.1 34.32,22.44 U$4.25
  Bottom 0.61: v23.82,34.83 28.99,34.83 29.97,35.81 29.97,39.24 30.61,39.88 34.62,39.88 34.75,39.75
  Bottom 1.27: J2.P$1 34.75,39.75 34.75,35.22 v34.58,35.05 | J9.P$1 34.75,13.32 v34.73,13.34
  other vias: 33.83,35.05 33.83,29.72 34.75,29.72 37.41,33.45 38.02,32.84 37.41,34.98 37.41,34.21 33.99,18.67 34.75,18.67 33.99,13.34 37.49,14.94 37.49,14.17 37.49,13.41 37.95,15.54 34.72,22.84 23.82,33.99 23.82,36.5 23.82,35.67
  pour Top (no thermals): 33.6,29.41 33.6,30.78 34.98,30.78 34.98,29.41
  pour Top (no thermals): 33.6,33.99 33.6,35.36 34.98,35.36 34.98,33.99
  pour Bottom: 33.6,29.41 33.6,35.36 39.17,35.36 39.17,32.38 35.13,29.41
  pour Top (no thermals): 39.78,36.27 37.03,36.27 37.03,33.22 37.95,32.31 39.78,32.31
  pour Top (no thermals): 33.68,17.6 33.68,18.97 35.05,18.97 35.05,17.6
  pour Top (no thermals): 33.68,14.48 33.68,13.03 35.05,13.03 35.05,14.48
  pour Bottom: 39.24,13.03 33.68,13.03 33.68,18.97 35.05,18.97 39.24,16.08
  pour Top (no thermals): 39.55,16 39.55,12.19 37.03,12.19 37.03,15.39 37.64,16
  pour Bottom: 33.6,29.41 33.68,18.97 35.05,18.97 36.27,18.21 36.27,30.25 35.13,29.41
  pour Top (no thermals): 21.38,36.89 24.2,36.89 24.2,33.61 21.38,33.61
  pour Bottom: 24.2,36.89 24.2,33.61 22.75,33.61 22.75,36.89

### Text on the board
tPlace: GND | V+ | usb < - > tmc | A1 | A2 | B1 | B2 | mkstepper v0.1 | V+ | NP1 | GND | V+
bPlace: one at a time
